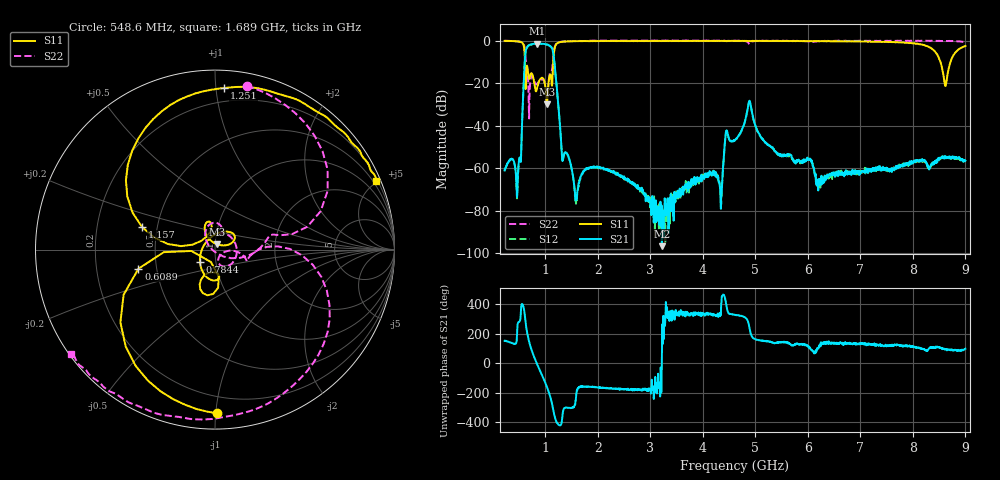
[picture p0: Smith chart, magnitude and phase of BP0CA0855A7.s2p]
!Agilent Technologies,E8358A,US41080443,A.07.50.56
!Agilent E8358A: A.07.50.56
!Date: Thursday, November 09, 2017 08:32:26
!Correction: S11(Full 2 Port(1,2))
!S21(Full 2 Port(1,2))
!S12(Full 2 Port(1,2))
!S22(Full 2 Port(1,2))
!S2P File: Measurements: S11, S21, S12, S22:
# Hz S  dB  R 50
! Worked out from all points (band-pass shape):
!   1601 points, 225 MHz to 9 GHz, reference 50 ohm
!   highest |S21| = -1.33 dB at 844.7 MHz (marker M1); lowest = -96.6 dB at 3.219 GHz (marker M2)
!   |S21| within 3 dB of the highest: 631.3 MHz to 1.139 GHz (507.6 MHz wide, 57.4 % of centre)
!   lowest |S11| = -29.9 dB at 1.031 GHz (marker M3), VSWR 1.07, Z = 50.9 + j3.09 ohm
!   |S11| at or under -10 dB: 613.1 MHz to 1.15 GHz (536.9 MHz wide, 60.9 % of centre); 8.525 GHz to 8.716 GHz (190.9 MHz wide, 2.21 % of centre)
!   |S22| runs from -36.5 to 0.1 dB; largest |S21 - S12| = 0.016
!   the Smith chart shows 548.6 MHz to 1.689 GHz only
!   S11 on the Smith chart (normalised r, x): 548.6 MHz: 0.09, -1.01; 608.9 MHz: 0.39, -0.10; 784.4 MHz: 0.84, -0.12; 1.157 GHz: 0.41, +0.13; 1.251 GHz: 0.11, +1.05; 1.689 GHz: 0.30, +4.88
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2.25e8  -0.08 -19.9  -60.96 151.2  -61.06 152.8  -0.04 155.1
4.8825e8  -0.37 -63.5  -58.99 -83.4  -59.40 -82.3  -0.32 104.9
5.485781e8  -0.80 -89.4  -45.19 36.6  -45.25 36.7  -0.64 79.0
6.089062e8  -7.14 -166.0  -9.58 -32.4  -9.71 -32.2  -4.06 19.9
6.856875e8  -17.74 -102.0  -2.10 154.2  -2.25 154.4  -31.54 -59.7
7.844062e8  -19.21 -139.5  -1.45 45.1  -1.61 45.2  -18.60 70.5
8.447344e8  -22.28 99.5  -1.33 -6.9  -1.49 -6.8  -20.17 66.8
1.031203e9  -29.91 71.5  -1.72 -160.2  -1.87 -160.1  -27.48 -43.9
1.157344e9  -7.40 162.7  -6.76 33.4  -6.93 33.5  -6.27 -3.7
1.250578e9  -0.90 86.8  -30.99 -54.9  -31.09 -54.7  -0.80 -73.5
1.568672e9  -0.25 32.1  -72.52 80.6  -73.84 92.7  -0.10 -134.1
1.689328e9  -0.21 23.1  -63.00 -155.3  -63.20 -158.9  -0.09 -144.0
3.153656e9  -0.14 -27.3  -82.12 -154.1  -85.20 -76.7  0.12 -172.0
3.219469e9  -0.15 -28.6  -96.57 57.3  -79.41 -154.9  0.10 -172.5
4.332797e9  -0.12 -46.8  -70.54 -19.0  -70.73 -28.2  0.07 177.3
4.447969e9  -0.21 -48.1  -42.24 30.3  -42.26 29.4  -0.11 175.7
4.6125e9  -0.06 -49.8  -46.60 -33.5  -46.62 -32.9  0.02 172.8
4.892203e9  -0.16 -53.1  -28.28 -129.6  -28.50 -129.1  -1.60 170.4
6.076828e9  -0.18 -68.9  -56.30 90.7  -56.88 89.8  -0.60 143.5
7.541156e9  -0.64 -113.5  -60.46 120.1  -61.57 119.3  -0.10 116.2
8.511891e9  -9.17 143.2  -55.28 103.3  -55.17 105.5  -0.10 102.2
9e9  -2.49 -112.1  -56.39 97.8  -56.64 94.5  -0.69 93.9
